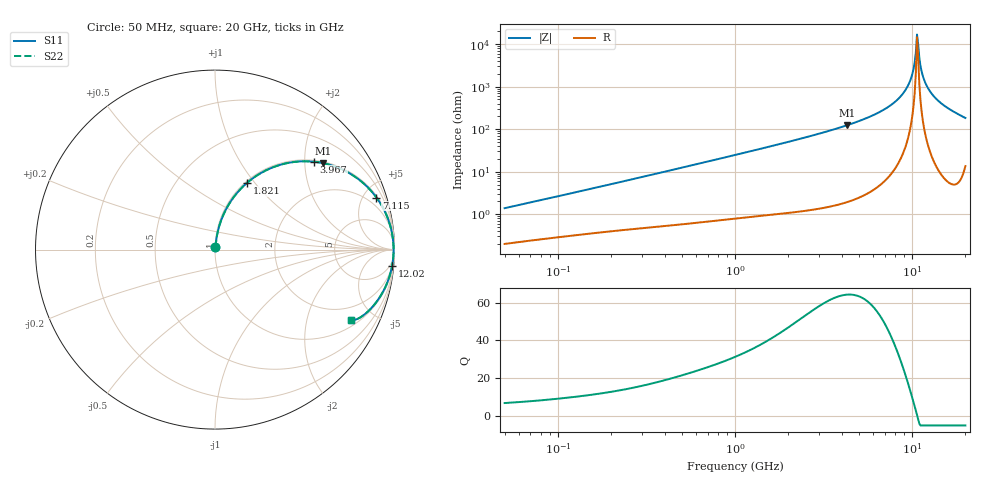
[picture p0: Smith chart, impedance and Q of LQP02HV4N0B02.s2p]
!Murata Part Number: LQP02HV4N0B02
!These Parameters are Measured in Series Mode Connection
!  o--[Z]--o
!Port1  Port2
!  o-------o
!Freq. Start=50[MHz] Stop=20[GHz], 401[Steps]
# Hz S RI R 50
!Freq.(Hz) S11(Real) S11(Imag) S21(Real) S21(Imag) S12(Real) S12(Imag) S22(Real) S22(Imag)
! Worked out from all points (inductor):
!   401 points, 50 MHz to 20 GHz, reference 50 ohm
!   read as one part in series: L = 4.3 nH near 51.52 MHz
!   highest Q = 64.2 at 4.276 GHz (marker M1), where L = 4.58 nH
!   self-resonance near 10.66 GHz
!   S11 on the Smith chart (normalised r, x): 50 MHz: 1.00, +0.03; 1.821 GHz: 1.02, +0.91; 3.967 GHz: 1.03, +2.23; 7.115 GHz: 1.13, +6.16; 12.02 GHz: 2, -22; 20 GHz: 1.27, -3.67
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5e7  0.00219 0.0137  0.9978 -0.0137  0.9978 -0.0137  0.00219 0.0137
1.364002e8  0.00456 0.035  0.9954 -0.035  0.9954 -0.035  0.00456 0.035
3.721004e8  0.0135 0.0912  0.9865 -0.0912  0.9865 -0.0912  0.0135 0.0912
1e9  0.0641 0.2294  0.9359 -0.2294  0.9359 -0.2294  0.0641 0.2294
1.820564e9  0.1775 0.371  0.8225 -0.371  0.8225 -0.371  0.1775 0.371
2.728004e9  0.3362 0.4635  0.6638 -0.4635  0.6638 -0.4635  0.3362 0.4635
3.967106e9  0.5525 0.4895  0.4475 -0.4895  0.4475 -0.4895  0.5525 0.4895
4.275624e9  0.6008 0.482  0.3992 -0.482  0.3992 -0.482  0.6008 0.482
5.683258e9  0.7815 0.405  0.2185 -0.405  0.2185 -0.405  0.7815 0.405
7.114996e9  0.8996 0.2902  0.1004 -0.2902  0.1004 -0.2902  0.8996 0.2902
7.442007e9  0.9186 0.2623  0.0814 -0.2623  0.0814 -0.2623  0.9186 0.2623
8.516016e9  0.9638 0.1711  0.0362 -0.1711  0.0362 -0.1711  0.9638 0.1711
9.457416e9  0.9856 0.0942  0.0144 -0.0942  0.0144 -0.0942  0.9856 0.0942
1.004137e10  0.9924 0.0489  0.00763 -0.0489  0.00763 -0.0489  0.9924 0.0489
1.050288e10  0.9947 0.0145  0.00532 -0.0145  0.00532 -0.0145  0.9947 0.0145
1.066139e10  0.9949 0.00298  0.00508 -0.00298  0.00508 -0.00298  0.9949 0.00298
1.098561e10  0.9946 -0.02  0.00542 0.02  0.00542 0.02  0.9946 -0.02
1.131968e10  0.9932 -0.043  0.00683 0.043  0.00683 0.043  0.9932 -0.043
1.201863e10  0.9871 -0.0887  0.0129 0.0887  0.0129 0.0887  0.9871 -0.0887
1.295331e10  0.9736 -0.1448  0.0264 0.1448  0.0264 0.1448  0.9736 -0.1448
1.460232e10  0.9384 -0.2302  0.0616 0.2302  0.0616 0.2302  0.9384 -0.2302
2e10  0.7561 -0.3941  0.2439 0.3941  0.2439 0.3941  0.7561 -0.3941
